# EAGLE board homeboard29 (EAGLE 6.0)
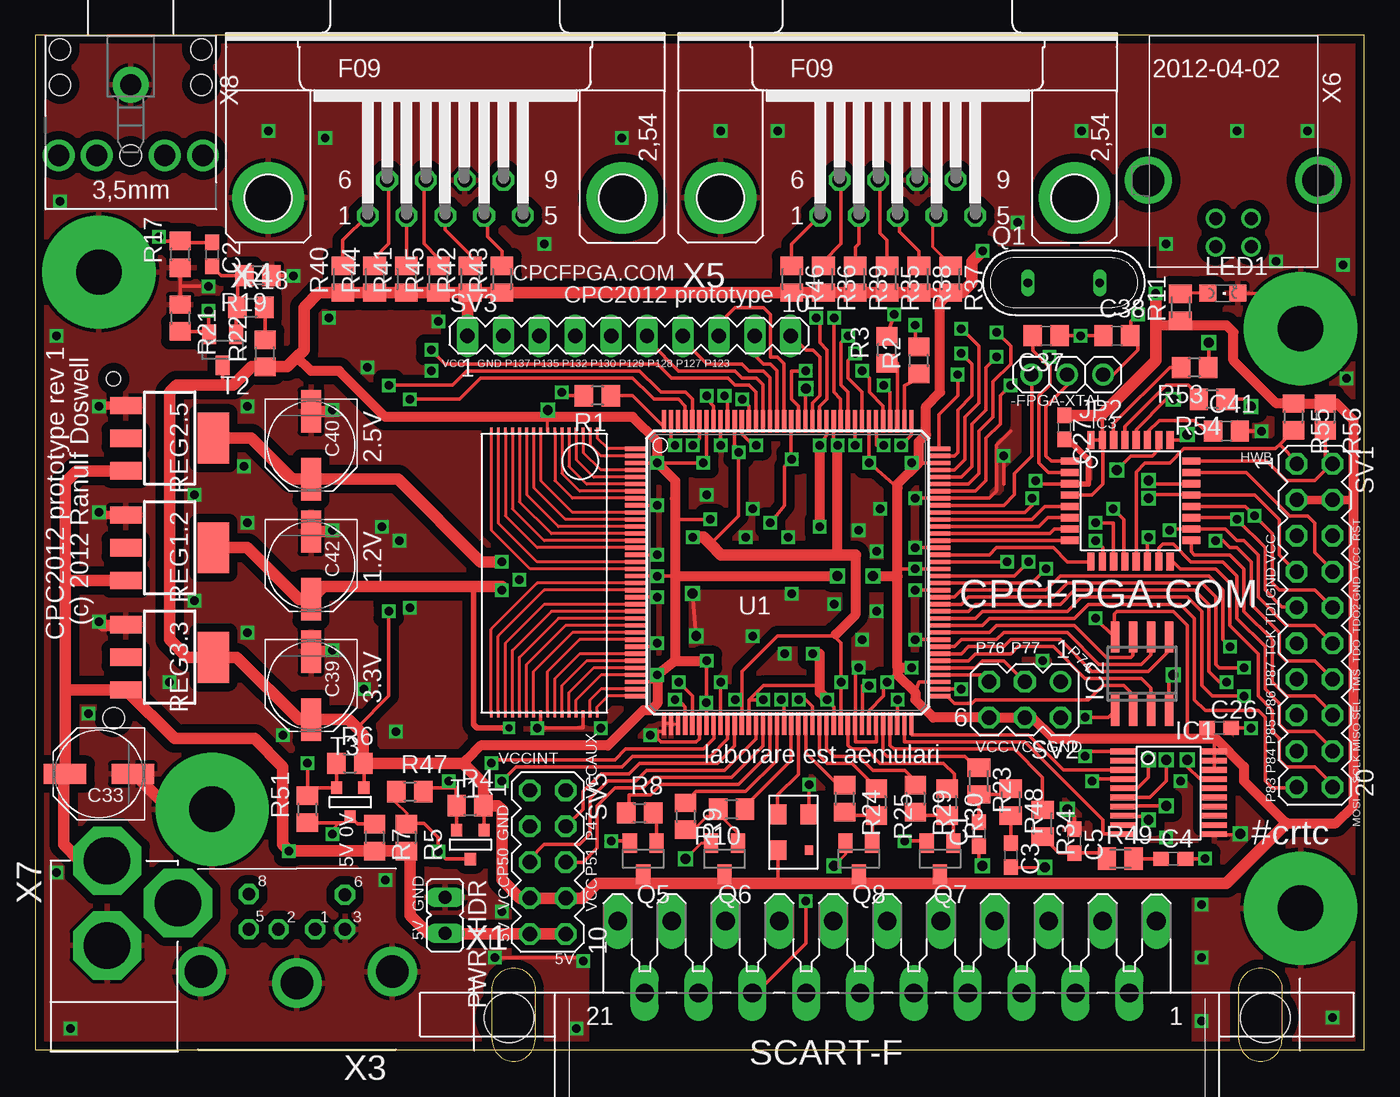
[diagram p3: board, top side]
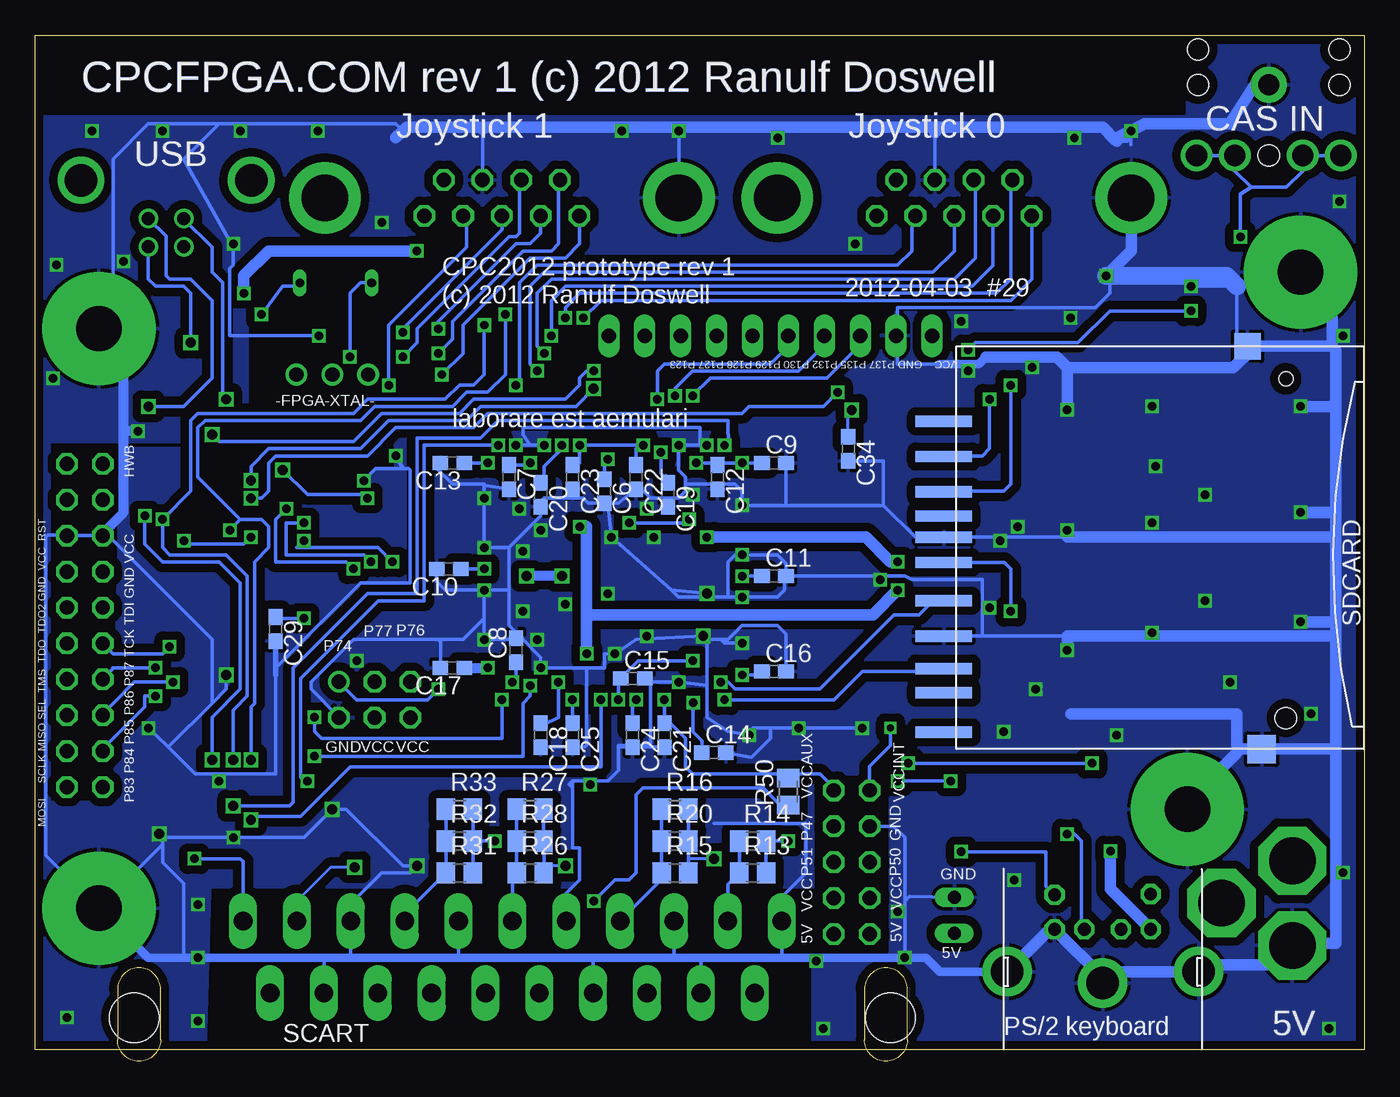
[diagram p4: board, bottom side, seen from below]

Size 94 x 72.58 mm. Coordinates in mm from the lower left corner, seen from the top.
Outline: 0,0.83 94,0.83 94,72.58 0,72.58 0,0.83
Copper layers (1*16): Top 0.0356mm / dielectric 1.5011mm / Bottom 0.0356mm
Design rules: minimum track width 7mil, minimum drill 15mil, track to track 7mil, track to pad 7mil, pad to pad 7mil, via to via 7mil, smd to smd 7mil, copper to edge 15mil, drill to drill 15mil, minimum pad ring 7mil, minimum via ring 7mil, stop-mask expansion 4mil, vias tented up to drill 0mil, thermal gap 10mil
Net classes: 1 power: width 0.6 mm, drill 1.1 mm, clearance 0.4 mm; 2 gnd: width 0.305 mm, drill 0.508 mm, clearance 0.152 mm

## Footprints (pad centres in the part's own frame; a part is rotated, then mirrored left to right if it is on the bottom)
C0603 = smd 1.1 x 1: 1 -0.85,0; 2 0.85,0
PANASONIC_D = smd 3 x 1.4: + 2.4,0; - -2.4,0
C0805 = smd 1.3 x 1.5: 1 -0.95,0; 2 0.95,0
VO20 = smd 0.4 x 1.8: 1 5.85,6.15; 2 5.2,6.15; 3 4.55,6.15; 4 3.9,6.15; 5 3.25,6.15; 6 2.6,6.15; 7 1.95,6.15; 8 1.3,6.15; 9 0.65,6.15; 10 0,6.15; 11 0,-0.3; 12 0.65,-0.3; 13 1.3,-0.3; 14 1.95,-0.3; 15 2.6,-0.3; 16 3.25,-0.3; 17 3.9,-0.3; 18 4.55,-0.3; 19 5.2,-0.3; 20 5.85,-0.3
SO-08 = smd 0.6 x 2.2: 1 -1.905,-2.6; 2 -0.635,-2.6; 3 0.635,-2.6; 4 1.905,-2.6; 5 1.905,2.6; 6 0.635,2.6; 7 -0.635,2.6; 8 -1.905,2.6
TQFP32-08 = smd 1.27 x 0.508: 1 -4.293,2.8; 2 -4.293,2; 3 -4.293,1.2; 4 -4.293,0.4; 5 -4.293,-0.4; 6 -4.293,-1.2; 7 -4.293,-2; 8 -4.293,-2.8; 17 4.293,-2.8; 18 4.293,-2; 19 4.293,-1.2; 20 4.293,-0.4; 21 4.293,0.4; 22 4.293,1.2; 23 4.293,2; 24 4.293,2.8 | smd 0.508 x 1.27: 9 -2.8,-4.293; 10 -2,-4.293; 11 -1.2,-4.293; 12 -0.4,-4.293; 13 0.4,-4.293; 14 1.2,-4.293; 15 2,-4.293; 16 2.8,-4.293; 25 2.8,4.293; 26 2,4.293; 27 1.2,4.293; 28 0.4,4.293; 29 -0.4,4.293; 30 -1.2,4.293; 31 -2,4.293; 32 -2.8,4.293
1X03 = drill 1.016: 1 -2.54,0; 2 0,0; 3 2.54,0
CHIPLED_0805 = smd 1.2 x 1.2: A 0,-1.05; C 0,1.05
JP1 = drill 0.914 long: 1 0,-1.27; 2 0,1.27
QS = drill 0.61 long: 1 -2.54,0; 2 2.54,0
SOT23 = smd 1 x 1.4: 1 -0.95,-1.1; 2 0.95,-1.1; 3 0,1.1
R0805 = smd 1.3 x 1.5: 1 -0.95,0; 2 0.95,0
M0805 = smd 1.3 x 1.6: 1 -0.95,0; 2 0.95,0
SOT223 = smd 1.219 x 2.235: 1 -2.311,-3.099; 2 0,-3.099; 3 2.311,-3.099 | smd 3.6 x 2.2: 4 0,3.099
MA10-2 = drill 1.016 octagon: 1 -11.43,-1.27; 2 -11.43,1.27; 3 -8.89,-1.27; 4 -8.89,1.27; 5 -6.35,-1.27; 6 -6.35,1.27; 7 -3.81,-1.27; 8 -3.81,1.27; 9 -1.27,-1.27; 10 -1.27,1.27; 11 1.27,-1.27; 12 1.27,1.27; 13 3.81,-1.27; 14 3.81,1.27; 15 6.35,-1.27; 16 6.35,1.27; 17 8.89,-1.27; 18 8.89,1.27; 19 11.43,-1.27; 20 11.43,1.27
MA03-2 = drill 1.016: 1 -2.54,-1.27 | drill 1.016 octagon: 2 -2.54,1.27; 3 0,-1.27; 4 0,1.27; 5 2.54,-1.27; 6 2.54,1.27
MA10-1 = drill 1.016 long: 1 -11.43,0; 2 -8.89,0; 3 -6.35,0; 4 -3.81,0; 5 -1.27,0; 6 1.27,0; 7 3.81,0; 8 6.35,0; 9 8.89,0; 10 11.43,0
MA05-2 = drill 1.016 octagon: 1 -5.08,-1.27; 2 -5.08,1.27; 3 -2.54,-1.27; 4 -2.54,1.27; 5 0,-1.27; 6 0,1.27; 7 2.54,-1.27; 8 2.54,1.27; 9 5.08,-1.27; 10 5.08,1.27
SOT-23 = smd 0.787 x 0.889: 1 0.025,-1.016; 2 -0.94,1.016; 3 0.991,1.016
TQ144 = smd 1.6 x 0.3: P1 -10.7,8.75; P2 -10.7,8.25; P3 -10.7,7.75; P4 -10.7,7.25; P5 -10.7,6.75; P6 -10.7,6.25; P7 -10.7,5.75; P8 -10.7,5.25; P9 -10.7,4.75; P10 -10.7,4.25; P11 -10.7,3.75; P12 -10.7,3.25; P13 -10.7,2.75; P14 -10.7,2.25; P15 -10.7,1.75; P16 -10.7,1.25; P17 -10.7,0.75; P18 -10.7,0.25; P19 -10.7,-0.25; P20 -10.7,-0.75; P21 -10.7,-1.25; P22 -10.7,-1.75; P23 -10.7,-2.25; P24 -10.7,-2.75; P25 -10.7,-3.25; P26 -10.7,-3.75; P27 -10.7,-4.25; P28 -10.7,-4.75; P29 -10.7,-5.25; P30 -10.7,-5.75; P31 -10.7,-6.25; P32 -10.7,-6.75; P33 -10.7,-7.25; P34 -10.7,-7.75; P35 -10.7,-8.25; P36 -10.7,-8.75; P73 10.7,-8.75; P74 10.7,-8.25; P75 10.7,-7.75; P76 10.7,-7.25; P77 10.7,-6.75; P78 10.7,-6.25; P79 10.7,-5.75; P80 10.7,-5.25; P81 10.7,-4.75; P82 10.7,-4.25; P83 10.7,-3.75; P84 10.7,-3.25; P85 10.7,-2.75; P86 10.7,-2.25; P87 10.7,-1.75; P88 10.7,-1.25; P89 10.7,-0.75; P90 10.7,-0.25; P91 10.7,0.25; P92 10.7,0.75; P93 10.7,1.25; P94 10.7,1.75; P95 10.7,2.25; P96 10.7,2.75; P97 10.7,3.25; P98 10.7,3.75; P99 10.7,4.25; P100 10.7,4.75; P101 10.7,5.25; P102 10.7,5.75; P103 10.7,6.25; P104 10.7,6.75; P105 10.7,7.25; P106 10.7,7.75; P107 10.7,8.25; P108 10.7,8.75 | smd 0.3 x 1.6: P37 -8.75,-10.7; P38 -8.25,-10.7; P39 -7.75,-10.7; P40 -7.25,-10.7; P41 -6.75,-10.7; P42 -6.25,-10.7; P43 -5.75,-10.7; P44 -5.25,-10.7; P45 -4.75,-10.7; P46 -4.25,-10.7; P47 -3.75,-10.7; P48 -3.25,-10.7; P49 -2.75,-10.7; P50 -2.25,-10.7; P51 -1.75,-10.7; P52 -1.25,-10.7; P53 -0.75,-10.7; P54 -0.25,-10.7; P55 0.25,-10.7; P56 0.75,-10.7; P57 1.25,-10.7; P58 1.75,-10.7; P59 2.25,-10.7; P60 2.75,-10.7; P61 3.25,-10.7; P62 3.75,-10.7; P63 4.25,-10.7; P64 4.75,-10.7; P65 5.25,-10.7; P66 5.75,-10.7; P67 6.25,-10.7; P68 6.75,-10.7; P69 7.25,-10.7; P70 7.75,-10.7; P71 8.25,-10.7; P72 8.75,-10.7; P109 8.75,10.7; P110 8.25,10.7; P111 7.75,10.7; P112 7.25,10.7; P113 6.75,10.7; P114 6.25,10.7; P115 5.75,10.7; P116 5.25,10.7; P117 4.75,10.7; P118 4.25,10.7; P119 3.75,10.7; P120 3.25,10.7; P121 2.75,10.7; P122 2.25,10.7; P123 1.75,10.7; P124 1.25,10.7; P125 0.75,10.7; P126 0.25,10.7; P127 -0.25,10.7; P128 -0.75,10.7; P129 -1.25,10.7; P130 -1.75,10.7; P131 -2.25,10.7; P132 -2.75,10.7; P133 -3.25,10.7; P134 -3.75,10.7; P135 -4.25,10.7; P136 -4.75,10.7; P137 -5.25,10.7; P138 -5.75,10.7; P139 -6.25,10.7; P140 -6.75,10.7; P141 -7.25,10.7; P142 -7.75,10.7; P143 -8.25,10.7; P144 -8.75,10.7
GNDHOLE = drill 3.2 pad 8: GND 0,0
OSC_7C = smd 0.7 x 0.6: ENA -1.27,-1.1 | smd 1.4 x 1.2: GND 1.27,-1.1; OUT 1.27,1.1; VDD -1.27,1.1
SDCARD-NOHOLE = smd 0.8 x 4 bottom: 1 7.8,0.99; 2 10.3,0.99; 3 13.5,0.99; 4 15.3,0.99; 5 18,0.99; 6 20.5,0.99; 7 22.8,0.99; 8 24.5,0.99; 9 5.3,0.99; CD 12,0.99; WP 27.3,0.99 | smd 2.032 x 2.032 bottom: MT1 28.5,-21.5 | smd 1.9 x 1.9 bottom: MT3 0,-20.5 | hole 1.5: 26.3,-23.21 | hole 1: 2.3,-23.21
TSOP32 = smd 0.5 x 0.2: P1 -9.75,3.75; P2 -9.75,3.25; P3 -9.75,2.75; P4 -9.75,2.25; P5 -9.75,1.75; P6 -9.75,1.25; P7 -9.75,0.75; P8 -9.75,0.25; P9 -9.75,-0.25; P10 -9.75,-0.75; P11 -9.75,-1.25; P12 -9.75,-1.75; P13 -9.75,-2.25; P14 -9.75,-2.75; P15 -9.75,-3.25; P16 -9.75,-3.75; P17 10.25,-3.75; P18 10.25,-3.25; P19 10.25,-2.75; P20 10.25,-2.25; P21 10.25,-1.75; P22 10.25,-1.25; P23 10.25,-0.75; P24 10.25,-0.25; P25 10.25,0.25; P26 10.25,0.75; P27 10.25,1.25; P28 10.25,1.75; P29 10.25,2.25; P30 10.25,2.75; P31 10.25,3.25; P32 10.25,3.75
SCART-CLIP = drill 1.321 long: 1 19.05,5.08; 2 17.145,0; 3 15.24,5.08; 4 13.335,0; 5 11.43,5.08; 6 9.525,0; 7 7.62,5.08; 8 5.715,0; 9 3.81,5.08; 10 1.905,0; 11 0,5.08; 12 -1.905,0; 13 -3.81,5.08; 14 -5.715,0; 15 -7.62,5.08; 16 -9.525,0; 17 -11.43,5.08; 18 -13.335,0; 19 -15.24,5.08; 20 -17.145,0; 21 -19.05,5.08 | hole 3.5: 26.75,-1.75; -26.75,-1.75
M_DIN6 = drill 0.9 pad 1.422 octagon: 1 -1.3,-3.75; 2 1.3,-3.75; 3 -3.4,-3.75; 5 3.4,-3.75; 6 -3.4,-6.2; 8 3.4,-6.25 | drill 2.3 pad 3.5: SH1 6.8,-0.75; SH2 0,0.05; SH3 -6.75,-0.75
F09HP = drill 1.016 octagon: 1 -5.486,-1.27; 2 -2.743,-1.27; 3 0,-1.27; 4 2.743,-1.27; 5 5.486,-1.27; 6 -4.115,1.27; 7 -1.372,1.27; 8 1.372,1.27; 9 4.115,1.27 | drill 3.302 pad 5.08: G1 -12.522,0; G2 12.522,0
85-32004-10X = drill 0.92 pad 1.27: 1 4.71,-1.25; 2 4.71,1.25; 3 2.71,1.25; 4 2.71,-1.25 | drill 2.3 pad 3: M1 0,6.02; M2 0,-6.02
DC-21MM = drill 3.302 pad 4.826 octagon: 1 -5.08,-3.353; 2 -0.076,-6.35; 3 -0.076,-0.356
20-0137 = drill 1.5 pad 2.54: 1 -5,0 | drill 1.5: 2 0,5.1; 3 0,2.4; 4 0,-2.4; 5 0,-5.1 | hole 1.5: -5,5; -5,-5; 0,0; -7.5,5; -7.5,-5

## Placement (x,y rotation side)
C1  [C0603]  66.75,16.08 90 top
C2  100nF  [C0603]  12.5,57.08 270 top
C3  [C0603]  69,14.58 270 top
C4  [C0603]  80.5,14.33 0 top
C5  [C0603]  73.5,15.58 270 top
C6  100nF  [C0603]  53.75,40.33 270 bottom
C7  100nF  [C0603]  60.5,41.33 270 bottom
C8  100nF  [C0603]  60,29.08 90 bottom
C9  100nF  [C0603]  41.75,42.33 0 bottom
C10  100nF  [C0603]  64.75,34.83 180 bottom
C11  100nF  [C0603]  41.75,34.33 0 bottom
C12  100nF  [C0603]  45.75,41.33 270 bottom
C13  100nF  [C0603]  64.5,42.33 180 bottom
C14  100nF  [C0603]  46,21.83 0 bottom
C15  100nF  [C0603]  51.75,27.08 0 bottom
C16  100nF  [C0603]  41.75,27.58 0 bottom
C17  100nF  [C0603]  64.5,27.83 180 bottom
C18  100nF  [C0603]  58.25,23.08 270 bottom
C19  100nF  [C0603]  49.25,40.08 270 bottom
C20  100nF  [C0603]  58.25,40.08 270 bottom
C21  100nF  [C0603]  49.5,23.08 270 bottom
C22  100nF  [C0603]  51.5,41.33 270 bottom
C23  100nF  [C0603]  56,41.33 270 bottom
C24  100nF  [C0603]  51.75,23.08 270 bottom
C25  100nF  [C0603]  56,23.08 270 bottom
C26  100nF  [C0603]  83.75,23.58 0 top
C27  100nF  [C0603]  72.8,44.84 270 top
C29  100nF  [C0603]  77,30.58 270 bottom
C33  100u  [PANASONIC_D]  4.5,20.33 180 top
C34  100nF  [C0603]  36.5,43.33 270 bottom
C37  [C0805]  71.5,51.33 180 top
C38  [C0805]  76.5,51.33 0 top
C39  100u  [PANASONIC_D]  19.5,26.58 270 top
C40  100u  [PANASONIC_D]  19.5,43.58 270 top
C41  1uF  [C0805]  84.25,44.58 0 top
C42  100u  [PANASONIC_D]  19.5,35.08 270 top
IC1  XCF02S  [VO20]  83.09,16.06 90 top
IC2  25LC080SN  [SO-08]  78.28,27.41 0 top
IC3  ATMEGA32U2-TQFP  [TQFP32-08]  77.47,39.65 0 top
JP2  [1X03]  73,48.58 180 top
LED1  [CHIPLED_0805]  84,54.33 270 top
PWR_HDR  [JP1]  29,10.33 180 top
Q1  [QS]  72.75,55.08 0 top
Q5  BC848SMD  [SOT23]  43,14.33 180 top
Q6  BC848SMD  [SOT23]  48.75,14.33 180 top
Q7  BC848SMD  [SOT23]  64,14.33 180 top
Q8  BC848SMD  [SOT23]  58.25,14.33 180 top
R1  100  [R0805]  39.76,47.07 180 top
R2  100  [R0805]  62.5,49.58 90 top
R3  100  [R0805]  60.25,50.33 90 top
R4  1000  [R0805]  30.75,18.08 0 top
R5  1000  [R0805]  26.25,15.83 270 top
R6  1000  [R0805]  22.25,21.08 0 top
R7  1000  [R0805]  24,15.83 270 top
R8  2200  [R0805]  42.75,17.58 0 top
R9  2200  [R0805]  46,17.33 270 top
R10  1000  [R0805]  49.25,17.83 180 top
R11  [M0805]  81,53.33 90 top
R13  680  [R0805]  43.25,13.33 0 bottom
R14  2200  [R0805]  43.25,15.58 0 bottom
R15  270  [R0805]  48.75,13.33 0 bottom
R16  680  [R0805]  48.75,17.83 0 bottom
R17  10000  [R0805]  10.25,57.08 90 top
R18  4700  [R0805]  15.25,53.33 0 top
R19  10000  [R0805]  15.75,55.58 180 top
R20  4700  [R0805]  48.75,15.58 0 bottom
R21  47000  [R0805]  10.25,52.58 270 top
R22  1000  [R0805]  16.25,50.08 90 top
R23  [M0805]  66.75,19.83 270 top
R24  2200  [R0805]  57.25,18.58 270 top
R25  1000  [R0805]  59.5,18.33 270 top
R26  270  [R0805]  59,13.33 0 bottom
R27  680  [R0805]  59,17.83 0 bottom
R28  4700  [R0805]  59,15.58 0 bottom
R29  2200  [R0805]  62.25,18.58 270 top
R30  1000  [R0805]  64.5,18.33 270 top
R31  270  [R0805]  64,13.33 0 bottom
R32  680  [R0805]  64,15.58 0 bottom
R33  4700  [R0805]  64,17.83 0 bottom
R34  [M0805]  71.25,16.83 270 top
R35  [M0805]  60.25,55.33 270 top
R36  [M0805]  55.75,55.33 270 top
R37  [M0805]  64.75,55.33 270 top
R38  [M0805]  62.5,55.33 270 top
R39  [M0805]  58,55.33 270 top
R40  [M0805]  21.75,55.33 90 top
R41  [M0805]  26.25,55.33 90 top
R42  [M0805]  30.75,55.33 90 top
R43  [M0805]  33,55.33 90 top
R44  [M0805]  24,55.33 90 top
R45  [M0805]  28.5,55.33 90 top
R46  [M0805]  53.5,55.33 270 top
R47  270  [R0805]  26.5,19.08 0 top
R48  [M0805]  69,18.33 270 top
R49  [M0805]  76.75,14.33 0 top
R50  2k2  [M0805]  40.75,19.08 90 bottom
R51  270  [R0805]  19.25,17.83 90 top
R53  22  [R0805]  82,49.08 180 top
R54  22  [R0805]  83.25,46.83 180 top
R55  4700  [R0805]  89,45.58 270 top
R56  4700  [R0805]  91.25,45.58 270 top
REG1.2  1.2V  [SOT223]  9.5,36.33 270 top
REG2.5  2.5V  [SOT223]  9.5,44.08 270 top
REG3.3  3.3V  [SOT223]  9.5,28.58 270 top
SV1  [MA10-2]  90.5,30.83 270 top
SV2  [MA03-2]  70,25.58 180 top
SV3  [MA10-1]  42,51.33 0 top
SV5  [MA05-2]  36.25,14.08 270 top
T1  BSS138  [SOT-23]  30.75,15.33 0 top
T2  BC848  [SOT23]  13.25,50.33 180 top
T3  BSS138  [SOT-23]  22.25,18.33 0 top
U1  XC3S400TQ144  [TQ144]  53.22,34.58 0 top
U$1  GNDHOLE  [GNDHOLE]  12.5,17.83 0 top
U$2  TXO_7C  [OSC_7C]  53.62,16.2 90 top
U$3  SDMMCNOHOLE  [SDCARD-NOHOLE]  28.75,50.58 270 top
U$6  AS6C4008  [TSOP32]  36,34.83 270 top
U$7  GNDHOLE  [GNDHOLE]  4.5,55.83 0 top
U$8  GNDHOLE  [GNDHOLE]  89.5,51.83 0 top
U$9  GNDHOLE  [GNDHOLE]  89.5,10.83 0 top
X1  SCART-CLIP  [SCART-CLIP]  60.25,4.83 0 top
X3  [M_DIN6]  18.5,5.58 180 top
X4  [F09HP]  29,61.08 0 top
X5  [F09HP]  61,61.08 0 top
X6  MINI-USB_4P-85-32004-10X  [85-32004-10X]  84.75,62.33 270 top
X7  DC21MMX  [DC-21MM]  5,7.83 180 top
X8  STEREOJACK  [20-0137]  6.75,64.08 270 top

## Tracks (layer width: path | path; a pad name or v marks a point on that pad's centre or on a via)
AT_CLKO  (via drill 0.7)
  Top 0.254: v78.75,41.08 79,40.83 81.74,40.83 IC3.22 | U1.P124 54.47,47.55 v54.5,47.58
  Bottom 0.254: v78.75,41.08 78.75,42.08 77.5,43.33 71,43.33 69,45.33 63.5,45.33 62.5,46.33 55.75,46.33 v54.5,47.58
AT_RESET
  Top 0.254: IC3.24 87.13,42.45 88.5,41.08 90.5,41.08 91.75,42.33 | 91.75,42.33 91.75,42.28 SV1.2 | R56.2 91.25,42.83 91.75,42.33
B0
  Top 0.254: U1.P63 57.47,22.36 57.75,22.08 58.75,22.08 59.75,21.08 64.25,21.08 65,20.33 65,19.53 R30.1
B1
  Top 0.254: U1.P60 55.97,22.11 56.5,21.58 58.25,21.58 59.25,20.58 61.5,20.58 62.25,19.83 R29.1
CASIN  (via drill 0.6)
  Top 0.254: R21.2 12.1,51.63 T2.2 12.3,51.63 12.5,51.83 12.25,51.83 v12.25,53.08 | U1.P131 50.97,47.36 50.5,47.83 49.5,47.83 49,48.33 45,48.33 44,49.33 29,49.33 v28,50.33
  Bottom 0.254: v12.25,53.08 18,53.08 20.25,50.83 27.5,50.83 v28,50.33
CLK16
  Top 0.254: U1.P56 53.97,20.3 52.5,18.83 52.5,17.5 U$2.OUT
CLK_5V  (via drill 0.6)
  Top 0.2: 26.3,16.83 26.3,17.53 25.5,18.33 25.5,19.03 R47.1
  Top 0.254: T1.1 29.02,14.31 v28.5,14.83 28.5,15.83 27.5,16.83 26.3,16.83 R5.1
  Bottom 0.254: v28.5,14.83 22.5,14.83 22.5,12.38 X3.6
CSYNC
  Top 0.254: U1.P52 51.97,21.8 49.75,19.58 44.25,19.58 43.5,18.83 42,18.83 42,17.78 R8.1
DATA_5V  (via drill 0.6)
  Top 0.2: v21,16.08 21,16.38 21.5,16.88
  Top 0.254: R7.1 22.81,16.78 T3.1 21.84,16.88 21.5,16.88 R51.1
  Bottom 0.254: v21,16.08 20.5,16.08 20,15.58 20,9.53 X3.1
EMER_BOOT
  Top 0.254: SV1.1 89.23,42.4 88.05,43.58 88.05,43.68 | 88.05,43.68 R55.2 | IC3.13 77.87,41.7 78.5,42.33 80.25,42.33 81.25,43.33 87.7,43.33 88.05,43.68
EXP_A
  Top 0.254: U1.P47 49.47,22.3 48.25,21.08 42.75,21.08 42,20.33 40,20.33 38.75,19.08 38.75,17.83 37.52,16.6 SV5.4
EXP_B
  Top 0.254: U1.P50 50.97,22.8 48.75,20.58 43.25,20.58 42.5,19.83 40.5,19.83 39.25,18.58 39.25,16.08 38.5,15.33 36,15.33 34.98,14.31 SV5.5
EXP_C
  Top 0.254: U1.P51 51.47,22.3 49.25,20.08 43.75,20.08 43,19.33 41,19.33 39.75,18.08 39.75,15.08 38.75,14.08 SV5.6
EXTCLK
  Top 0.254: U1.P100 68.5,39.33 69.25,40.08 69.25,41.58 70.5,42.83 70.5,48.58 JP2.3
FL_DI
  Top 0.254: U1.P79 65.5,28.83 66,29.33 68.5,29.33 69,29.83 72.5,29.83 74.75,27.58 78.75,27.58 80.19,29.01 IC2.5
FL_DO
  Top 0.254: IC2.2 77.64,25.93 77,26.58 75.5,26.58 74.5,25.58 66.5,25.58 66.25,25.33 65,25.33 64.5,25.83 U1.P73
FL_HOLD
  Top 0.254: U1.P82 67.5,30.33 68,30.83 73.5,30.83 75.75,28.58 77.5,28.58 77.64,28.72 IC2.7
FL_SCLK
  Top 0.254: U1.P80 65,29.33 65.5,29.83 68,29.83 68.5,30.33 73,30.33 75.25,28.08 78.25,28.08 78.92,28.74 IC2.6
FL_SEL  (via drill 0.6)
  Top 0.254: v74.25,24.33 75.89,24.33 IC2.1 | v61,25.58 61,23.91 U1.P70
  Bottom 0.254: v74.25,24.33 74.25,23.33 73.75,22.83 61,22.83 v61,25.58
FL_WP
  Top 0.254: U1.P78 66,28.33 66.5,28.83 69,28.83 69.5,29.33 72,29.33 74.25,27.08 78.25,27.08 78.92,26.41 IC2.3
FPGA_AUDIO_LEFT
  Top 0.254: U1.P68 59.97,21.86 60.25,21.58 65.75,21.58 66.55,20.78 R23.1
FPGA_AUDIO_RIGHT
  Top 0.254: U1.P69 60.47,22.36 60.75,22.08 69.25,22.08 71.25,20.08 R34.1
G0
  Top 0.254: U1.P59 55.47,21.61 56,21.08 57.75,21.08 59,19.83 R25.1
G1
  Top 0.254: U1.P57 54.5,23.85 54.5,21.83 56.75,19.58 R24.1
GND  (via drill 0.6, 0.7)
  Top 0.2: U1.P37 U1.P38 U1.P39 | IC1.11 85.24,16.06 v85.25,16.08 | LED1.C 87,54.33 U$8.GND
  Top 0.254: U1.P9 v44,39.33 | U1.P22 v44,32.83 | U1.P16 v44,35.83 | U1.P81 v62.25,29.83 | U1.P88 v62.25,33.33 | U1.P94 v62.25,36.33 | U1.P117 57.97,43.86 v58,43.58 | v60,43.58 59.5,43.58 59.5,45.33 59.47,45.3 U1.P114 | U$6.P30 38.75,23.58 35.75,23.58 | U$6.P24 35.75,23.58 | 35.75,23.58 v35.5,23.58 | 44,23.33 v43.5,23.08 | U1.P29 43.75,29.33 v44,29.58 | U1.P42 46.97,22.8 46.75,22.58 44.25,22.58 44,22.83 44,23.33 | U1.P67 59.5,23.88 59.5,22.58 58,22.58 58,23.91 | v58.25,27.83 58,27.83 58,23.91 | 58,23.91 U1.P64 | R17.1 10.25,56.08 | R21.1 10.25,54.83 | 10.25,54.83 10.25,56.08 | 10.25,56.08 10,56.33 | R19.1 v18.25,55.58 | v12.25,54.83 10.25,54.83 | v62.25,39.83 U1.P101 67.5,39.83 68,40.33 68,43.58 69,44.58 | C38.1 v73.95,51.33 C37.1 | v70.75,41.08 71,40.83 73.15,40.83 IC3.3 73.23,40.85 73.25,40.83 | U1.P37 44.47,23.86 44.5,23.83 44.5,23.33 44,23.33 | U1.P39 45.47,23.86 45.5,23.83 | 68.5,40.83 v68.5,42.83 | U1.P45 48.47,26.55 v48.5,26.83 | U1.P136 48.47,43.86 v48.5,43.58 | 7,20.33 C33.- | 46.97,45.3 U1.P139 46.97,44.05 v46.5,43.58 | U$2.GND 54.73,19.55 v54.75,19.58 | v46.75,30.08 v46.5,33.08 | C5.1 73.5,17.33 v73,17.83 | IC2.4 80.19,27.01 v80.5,27.33 | C26.2 v86,23.58 | C1.1 66.75,14.08 v67,13.83 | v86.75,44.58 85.25,44.58 | 85.25,44.58 85,44.83 | C41.2 85.25,44.58 | v32.5,7.33 38.5,7.33 v38.75,7.08
  Top 0.406: C27.2 73.09,43.99 74.5,42.58 74.5,40.83 73.25,40.83
  Top 0.6: 6,30.83 6.4,30.83 REG3.3.1
  Top 0.61: REG2.5.1 4.56,46.39 v4.5,46.33 | REG1.2.1 4.69,38.64 v4.5,38.83
  Top 0.8: C39.- 20.5,28.98 v21,29.08 | C42.- 21,37.48 v21,37.58 | C40.- 21,45.98 v21,46.08 | U$1.GND 9.5,17.83 7,20.33
  Top 0.813: 6,30.83 4.75,30.83 v4.5,31.08
  Bottom 0.2: 25.5,6.33 X3.SH3 | 22.25,9.33 X3.3 | 18.5,5.93 X3.SH2 | v85.25,16.08 85,15.83 | 85,14.08 85,14.33
  Bottom 0.254: v62.25,33.33 62.15,33.23 | 62.25,31.33 v62.25,29.83 60.1,29.83 C8.2 | 62.25,31.33 v62.25,33.33 | 47,43.58 v48.5,43.58 48.5,41.83 48,41.33 48,40.93 | 47,43.58 v46.5,43.58 | 56,39.83 55.25,39.83 54.9,39.48 C6.2 | v58,43.58 59,43.58 | 59,43.58 v60,43.58 | 34,39.33 34,42.48 C34.2 | 47,43.58 47,44.83 59.5,44.83 59.5,44.33 59,43.58 | 60.5,33.33 v62.25,33.33 | v44,32.83 45,32.83 45,35.33 44.5,35.83 v44,35.83 41.5,35.83 40.9,35.23 C11.2 32.5,34.33 32,34.08 27,34.08 27,30.08 | 60.5,36.33 v62.25,36.33 v62.25,39.83 62.25,40.83 | v35.5,23.58 42,23.58 | 42,23.58 43.25,23.58 v43.5,23.08 45,23.33 46.5,24.33 46.5,26.58 | U$3.6 27,30.08 | 27,30.08 21,30.08 | 21,37.08 U$3.3 31.75,37.08 34,39.33 | v44,29.58 45.25,29.58 45.5,29.83 | 56,19.83 56,15.08 55.5,15.08 55.5,12.83 56.5,11.83 56.44,11.77 X1.13 | v12.25,54.83 9,54.83 9,51.33 U$3.MT3 | 81,66.33 83.5,63.83 80,57.58 80,56.33 80.25,56.08 80.25,51.33 v73.95,51.33 | 81,66.33 68.5,66.33 68,65.83 | 85,15.33 85,15.83 75,15.83 v73,17.83 72,17.83 68,13.83 v67,13.83 67.5,13.33 69.5,13.33 71.68,11.15 X1.5 71.68,7.65 | 85,15.33 85,14.08 83.5,12.58 83.5,7.33 | 30,49.33 33,49.33 33,51.33 SV3.2 33,51.44 33,53.33 19,53.33 18,54.33 18,55.33 v18.25,55.58 | X5.G1 48.48,66.05 | X4.8 30.37,65.45 31,66.08 | X5.8 62.37,65.95 | 81,66.33 86,66.33 88.5,63.83 88.5,51.33 U$8.GND | 77,27.33 77,20.33 82.7,20.33 84.6,22.23 | SV2.2 72.54,24.37 74.5,26.33 74.5,26.83 71.5,29.83 65.5,29.83 | 65.5,29.83 63.75,29.83 62.25,31.33 | v70.75,41.08 69.91,41.91 68,41.91 | 68,41.91 67.59,41.91 67.5,41.83 67.5,33.83 71,33.83 77,27.83 | v68.5,42.83 68,41.91 | 52.4,22.23 C24.2 C21.2 52.65,22.23 52.75,22.33
  Bottom 0.254: 55,27.83 55,22.33 55.15,22.23 C25.2 C18.2 | 52.75,22.33 52.75,20.58 53.5,19.83 54.75,19.83 | 52.75,22.33 50.5,22.33 50.5,26.83 | C16.2 40.9,30.23 41.5,30.83 44,30.83 45,29.83 45.5,29.83 | C10.2 65.6,33.93 65,33.33 v62.25,33.33 | C17.2 65.35,29.68 65.5,29.83 | 62.25,40.83 64.5,40.83 65.6,41.93 65.6,42.23 65.5,42.33 C13.2 | C14.2 43.35,21.48 42,22.83 42,23.58 | 46.5,29.83 v46.75,30.08 51.5,29.83 v53,28.83 53.75,28.83 53.75,27.83 55,27.83 | 46.5,29.83 45.5,29.83 | C15.2 50.5,26.83 | 50.5,26.83 v48.5,26.83 46.5,26.58 | 46.5,26.58 46.5,29.83 | 41,34.33 41,33.33 41.5,32.83 48.5,32.83 49,33.33 | C9.2 40.9,39.43 41,39.33 | 41,39.33 v44,39.33 44,40.33 44.5,40.83 45.65,40.83 C12.2 46.1,40.83 47.9,40.83 48,40.93 | 34,39.33 41,39.33 | 55,27.83 v58.25,27.83 58.25,28.58 59.5,29.83 60,29.83 | C7.2 62.15,40.73 62.25,40.83 | C23.2 56,39.83 | 48,40.93 48,40.33 48.5,39.83 49.5,39.83 | 9,21.83 9,22.08 | 17.5,65.33 17.62,65.2 | SV5.3 33.29,16.62 32.5,15.83 32.5,11.33 | 32.5,11.33 v32.5,7.33 | PWR_HDR.1 32.18,11.65 32.5,11.33 | 84.6,22.23 81.5,25.33 | 81.5,25.33 80.5,26.33 v80.5,27.33 | v86,23.58 84.7,22.33 84.6,22.23 | C19.2 49.4,39.73 49.5,39.83 | v54.75,19.58 54.75,19.83 | 17.5,65.08 16.75,65.08 16.5,65.33 16.5,64.83 | 60.5,36.33 60.5,33.33 | 60.5,33.33 60.5,30.83 60,30.33 | 49.5,39.83 50.5,39.83 51.5,40.83 C22.2 52.75,39.48 C6.2 | C20.2 58.25,38.58 60.5,36.33 | 56,39.83 58,39.83 58.5,39.33 58,39.33 | 49,33.33 v53.25,37.08 53.5,39.23 C6.2 | v46.5,33.08 49,33.33 | 85,15.33 U$9.GND 93.25,14.58 93.25,37.08 93.11,37.22 91.81,37.22 SV1.6 SV1.5 | 41,7.33 41.2,7.53 X1.21 41.2,11.63 39.5,13.33 39.5,16.83 46,16.83 | X1.18 46.91,7.24 47,7.33
  Bottom 0.254: X1.17 48.82,7.51 49,7.33 | X1.14 54.53,7.29 54.5,7.33 | X1.9 64.06,7.39 64,7.33 | X1.4 73.58,7.24 73.5,7.33 | 81.5,25.33 81.5,29.83 89,37.33 | 89.25,37.33 89.25,37.08 | 54.75,19.83 56,19.83 | 56,19.83 56.25,19.58 56,19.33
  Bottom 0.406: 77,27.33 77,27.83 C29.2
  Bottom 0.6: 4.93,8.33 X7.3 | 25.5,6.33 30,6.33 31,7.33 v32.5,7.33 41,7.33 47,7.33 49,7.33 54.5,7.33 64,7.33 73.5,7.33 83.5,7.33 86,7.33 U$9.GND | 26.75,49.83 27.25,49.33 30,49.33
  Bottom 0.61: 2,36.83 2,37.08
  Bottom 0.7: 89.25,37.33 87.75,38.83 87.75,44.58 | 87.75,44.58 87.75,49.58 U$8.GND | v86.75,44.58 87.75,44.58
  Bottom 0.8: 2,30.83 2,36.83 2,38.83 | X3.SH3 22.25,9.33 | X3.3 18.5,5.93 | X3.SH2 17.7,6.33 X3.SH1 11.2,6.83 6.43,6.83 X7.3 | 30.37,65.7 30,66.08 | 30,66.08 18.5,66.08 17.62,65.2 17.5,65.08 | 2,30.08 21,30.08 v21,29.08 | 2,37.08 21,37.08 v21,37.58 | v21,46.08 21,49.08 | 7.5,22.33 7.5,22.08 9,22.08 9,24.58 20.75,24.58 | U$1.GND 12.5,18.33 9,21.83 | 2,46.33 2,50.33 2.25,50.58 | 2,46.33 2,38.83 | v4.5,46.33 2,46.33 | v4.5,38.83 2,38.83 | 2.5,31.08 2.25,31.08 2,30.83 | 2,30.83 2,30.08 | U$3.MT1 2,22.08 | 2,22.08 2,30.08 | 4.93,8.33 2,8.33 2,22.08 | U$3.MT3 2.25,50.58 | 2.25,50.58 2.25,52.58 U$7.GND | 21,49.08 9.25,49.08 8,50.33 | 26.75,49.83 21.75,49.83 21,49.08 | X4.G1 16.48,57.35 v18.25,55.58 | X8.1 7.75,69.08 9.5,66.33 15.5,66.33 17.5,65.33 | 30,66.08 31,66.08 48.5,66.08 | 48.5,66.08 62.5,66.08 | 62.5,66.08 67.75,66.08 68,65.83 68.5,65.33 | 62.37,65.95 62.5,66.08 | 48.48,66.05 48.5,66.08
  Bottom 0.813: U$3.MT1 9,22.08 | v4.5,31.08 2.5,31.08
  Bottom 1.27: v18.25,55.58 9.75,55.58 9,54.83
  other vias: 15,38.08 85,65.83 82.5,2.83 26.5,32.08 2.5,2.33 59.5,36.08 59.5,31.83 71.25,28.33 41.5,65.33 74,65.83 15,30.33 15,46.33 9.5,26.83 23.5,49.08 47.5,40.08 56.5,32.33 34.25,34.08 25.5,23.33 81,19.83 20.5,65.33 52.5,65.83 24.5,37.83 87.75,56.58 69.5,59.33 80,57.83 36,57.83 20.75,52.58 92.75,48.33 59.75,39.08 53.5,33.08 50.75,30.08 92.5,56.33 90,65.83 79.5,65.83 48.5,65.83 16.5,65.83 38.25,2.33 1.5,13.33 91.75,3.08 1.75,60.83 82.5,7.33 50.75,39.08 80,15.83 82.5,11.08 40,23.58 3.75,24.58 28,48.83 50.25,37.08 28.5,52.33 14.75,42.08 11.25,40.08 11.25,32.58 17.5,23.08 23.25,26.33 25.75,36.83 1.5,51.33 24.75,12.83 33,10.58 58.25,37.58 58.5,29.83
  pour Bottom (isolate 0.6): 0,72.83 12.5,72.83 12.5,66.83 94,66.83 94,16.33 93,16.33 93,43.83 79,43.83 79,57.33 66,57.33 66,51.33 68.5,51.33 68.5,41.83 70,41.83 71,40.83 76,40.83 76,43.33 88,43.33 88.5,12.33 56,12.33 56,19.83 54.5,19.83 54.5,26.33 53.5,26.33 53.5,19.83 51.5,19.83 51.5,12.33 39,12.33 39,20.33 0,20.33
  pour Bottom (isolate 0.6): -0.5,0.33 -0.5,23.33 33.5,23.33 33.5,7.33 39,7.33 39,0.83 82,0.83 81.5,18.33 94.5,18.33 94.5,0.83
  pour Top (isolate 0.6): 0,72.83 94.5,72.83 94.5,43.83 79.5,43.83 79.5,57.83 66.5,57.83 66.5,46.33 70,46.33 70,41.83 55.5,41.83 55.5,53.33 28.5,53.33 28.5,48.83 53.5,48.83 53.5,44.83 -0.5,44.83 -0.5,72.83
  pour Top (isolate 0.6): -0.5,1.33 -0.5,49.33 69,49.33 69,40.33 74.5,40.33 74.5,45.83 88,45.83 88,26.33 85,26.33 85,20.83 85.5,20.83 85.5,19.83 88,19.83 88,15.33 67.5,15.33 67.5,22.83 81,22.83 81,28.33 66,28.33 66,12.83 56.5,12.83 56.5,19.33 54.5,19.33 54.5,25.33 51,25.33 51,12.83 39,12.83 39,20.33 33.5,20.33 33.5,7.33 39,7.33 39,1.33
  pour Top (isolate 0.6): 94.5,0.83 94.5,17.83 82,17.83 82,0.83
HDR_MISO  (via drill 0.6)
  Top 0.254: v84.25,26.83 83.75,26.83 83,27.58 83,32.33 82,33.33 73.5,33.33 72.5,32.33 66.5,32.33 66,31.83 U1.P85
  Bottom 0.254: v84.25,26.83 87,26.83 88.5,25.33 88.97,24.83 89.23,24.57 SV1.15
HDR_MOSI
  Top 0.254: 89.07,19.4 89.25,19.58 | U1.P83 67,30.83 67.5,31.33 73.5,31.33 74.5,32.33 81,32.33 82,31.33 82,25.58 82.75,24.83 86.5,24.83 87,24.33 87,19.83 87.5,19.33 89,19.33 89.07,19.4 | SV1.19 89.07,19.4
HDR_SCLK  (via drill 0.6)
  Top 0.254: v85.5,25.83 83.25,25.83 82.5,26.58 82.5,31.83 81.5,32.83 74,32.83 73,31.83 67,31.83 66.5,31.33 U1.P84
  Bottom 0.254: v85.5,25.83 86.25,25.83 86.25,25.08 89.23,22.1 SV1.17
HDR_SEL  (via drill 0.6)
  Top 0.254: v85.5,27.83 83.75,27.83 83.5,28.08 83.5,32.83 82.5,33.83 73,33.83 72,32.83 66,32.83 65.5,32.33 U1.P86
  Bottom 0.254: v85.5,27.83 88.51,27.83 88.51,27.74 SV1.13
HDR_SPARE  (via drill 0.6)
  Top 0.254: v84.5,29.33 84,29.83 84,33.33 83,34.33 72.5,34.33 71.5,33.33 65.5,33.33 65,32.83 U1.P87
  Bottom 0.254: v84.5,29.33 85,28.83 88.5,28.83 SV1.11 89.25,29.58
JOY0_DOWN  (via drill 0.6)
  Top 0.254: U1.P118 57.47,47.36 57,47.83 57,50.83 v57.5,51.33 | R41.2 X4.2
  Bottom 0.254: v57.5,51.33 57.5,53.83 56.5,54.83 27.7,54.83 R41.2 X4.2
JOY0_FIRE1  (via drill 0.6)
  Top 0.254: U1.P116 58.47,47.36 57.5,48.33 57.5,49.58 v58,50.08 | R45.2 28.5,56.83 27.5,57.83 27.5,62.22 X4.7
  Bottom 0.254: v58,50.08 58.5,50.58 58.5,54.33 57.5,55.33 29,55.33 27.5,56.83 27.5,62.22 X4.7
JOY0_FIRE2  (via drill 0.6)
  Top 0.254: U1.P119 56.97,46.86 56.5,47.33 v56.5,52.58 | R44.2 24,56.83 25,57.83 25,62.23 X4.6
  Bottom 0.254: v56.5,52.58 56.5,53.33 55.5,54.33 26,54.33 25,55.33 25,62.23 X4.6
JOY0_LEFT  (via drill 0.6)
  Top 0.254: U1.P113 59.97,46.36 59,47.33 59,48.33 v58.5,48.83 | R42.2 30.75,57.08 29,58.83 X4.3
  Bottom 0.254: v58.5,48.83 59,49.33 59,54.83 58,55.83 30.5,55.83 29,57.33 X4.3
JOY0_RIGHT  (via drill 0.6)
  Top 0.254: U1.P112 60.47,47.36 v60,47.83 | R43.2 33,57.33 32,58.33 32,59.55 X4.4
  Bottom 0.254: v60,47.83 59.75,47.83 59.75,55.08 58.5,56.33 33,56.33 32,57.33 32,59.55 X4.4
JOY0_UP  (via drill 0.6)
  Top 0.254: U1.P122 55.47,46.3 56,46.83 56,50.33 55.5,50.83 55.5,52.33 v55.25,52.58 | R40.2 21.75,58.08 23.5,59.83 X4.1
  Bottom 0.254: v55.25,52.58 54,53.83 25,53.83 23.5,55.33 23.5,59.79 X4.1
JOY1_DOWN  (via drill 0.6)
  Top 0.254: U1.P105 65,41.83 65.75,42.58 65.75,45.58 66.75,46.58 66.75,50.58 v65.5,51.83 | R39.1 58,57.58 58.25,57.83 X5.2
  Bottom 0.254: X5.2 58.26,58.58 59.01,57.83 60,57.83 65.5,52.33 v65.5,51.83
JOY1_FIRE1  (via drill 0.6)
  Top 0.254: U1.P104 65.5,41.33 66.25,42.08 66.25,45.08 67.25,46.08 67.25,49.08 v68,49.83 | R35.1 60.25,58.08 59.75,58.58 59.75,62.22 X5.7
  Bottom 0.254: X5.7 59.75,62.22 59.75,58.58 60,58.33 60.5,58.33 67,51.83 67,50.83 v68,49.83
JOY1_FIRE2  (via drill 0.6)
  Top 0.254: R36.1 55.75,56.58 57,57.83 57,62.23 X5.6 | U1.P107 65,42.83 65.25,43.08 65.25,46.08 66.25,47.08 66.25,49.33 v65.5,50.08
  Bottom 0.254: X5.6 57,62.23 57,57.83 57.5,57.33 59.5,57.33 64.5,52.33 64.5,51.08 v65.5,50.08
JOY1_LEFT  (via drill 0.6)
  Top 0.254: U1.P103 66,40.83 66.75,41.58 66.75,44.58 67.75,45.58 67.75,48.08 69,49.33 69,50.58 v68,51.58 | R38.1 62.5,57.33 61.12,58.7 61.12,59.68 X5.3
  Bottom 0.254: 61,59.83 X5.3 61,58.83 68,51.83 v68,51.58
JOY1_RIGHT  (via drill 0.6)
  Top 0.2: R37.1 64.75,56.33 63.5,57.58 63.5,59.56 X5.4
  Top 0.254: U1.P102 66.5,40.33 67.25,41.08 67.25,44.08 68.25,45.08 68.25,47.08 v69,47.83
  Bottom 0.254: X5.4 63.5,59.56 63.5,57.58 69,52.08 v69,47.83
JOY1_UP  (via drill 0.6)
  Top 0.254: 55.5,59.83 X5.1 53.5,57.79 R46.1 | U1.P108 63.92,45.75 65.25,47.08 v65.25,48.58
  Bottom 0.254: X5.1 55.5,59.79 55.5,57.83 56.5,56.83 59,56.83 63.75,52.08 63.75,50.08 v65.25,48.58
N$1  (via drill 0.6)
  Top 0.254: U1.P135 48.97,46.86 v48.75,47.08
  Bottom 0.254: v48.75,47.08 48.75,47.58 47.5,48.83 40,48.83 38.25,50.58 38.25,51.27 SV3.4
N$2  (via drill 0.6)
  Top 0.254: U1.P132 50.47,46.36 v50,46.83
  Bottom 0.254: v50,46.83 50,48.83 49.5,49.33 42,49.33 41,50.33 41,51.08 40.75,51.33 SV3.5
N$3  (via drill 0.6)
  Top 0.254: U1.P137 47.97,46.36 47.5,46.83 v47.5,47.08
  Bottom 0.254: v47.5,47.08 46.25,48.33 38,48.33 35.5,50.83 35.5,51.18 SV3.3
N$4
  Top 0.254: U1.P130 51.47,47.86 51,48.33 50,48.33 49.5,48.83 45.5,48.83 43.5,50.83 43.5,51.1 SV3.6
N$5
  Top 0.254: U1.P129 51.97,48.36 51.5,48.83 50.5,48.83 50,49.33 47.5,49.33 46,50.83 46,51.08 45.75,51.33 SV3.7
N$6
  Top 0.254: U1.P128 52.47,48.86 52,49.33 51.5,49.33 51,49.83 51,51.33 SV3.9
N$7
  Top 0.254: U1.P127 52.97,49.36 52.5,49.83 52,49.83 52,52.83 51.5,53.33 49.5,53.33 48.5,52.33 48.5,51.48 SV3.8
N$8
  Top 0.254: 72.88,42.45 IC3.1 71.88,42.45 71.5,42.83 71.5,46.33 73,47.83 JP2.2
N$9
  Top 0.254: IC3.27 78.67,44.5 79.5,45.33 82,45.33 82.75,44.58 C41.1
N$10
  Top 0.2: LED1.A 81,54.33 R11.2
N$12  (via drill 0.6)
  Top 0.254: v71.75,49.83 71.75,49.08 | C37.2 70.55,50.28 71.75,49.08 | IC3.2 71.68,41.65 71,42.33 71,47.08 71.75,47.83 71.75,49.08
  Bottom 0.254: Q1.1 71,55.08 71.75,54.33 v71.75,49.83
N$14  (via drill 0.6)
  Top 0.254: v78,52.83 77.5,52.38 C38.2 78,51.28 78,50.33 76.25,48.58 JP2.1
  Bottom 0.254: Q1.2 75.54,54.83 76.5,54.83 v78,52.83
N$16
  Top 0.254: U1.P123 54.97,46.55 55.5,47.08 55.5,49.83 55,50.33 54.5,50.33 53.5,51.33 SV3.10
N$35
  Top 0.254: U1.P72 61.97,23.86 62,23.83 62,23.08 70.25,23.08 72.71,20.61 IC1.3
N$36  (via drill 0.7)
  Top 0.254: R53.1 83,49.13 v83,50.83
  Bottom 0.254: X6.2 86,55.33 85.5,54.83 83.5,54.83 83,54.33 v83,50.83
N$38
  Top 0.254: U1.P71 61.47,22.61 61.5,22.58 70,22.58 75.5,17.08 75.5,16.08 76.75,16.08 76.76,16.06 IC1.10
N$39
  Top 0.254: U1.P110 61.47,47.8 62.5,48.33 R2.1
N$40  (via drill 0.6, 0.7)
  Top 0.254: IC1.7 77,18.08 77,18.07 IC1.7 77.01,18.08 v80,18.08 | U1.P143 44.97,43.8 v45.25,43.58
  Bottom 0.254: v45.25,43.58 44.97,43.86 44.97,44.33 45,44.36 45,45.33 61.25,45.33 62.5,44.08 67,44.08 67,33.08 70.5,33.08 75.75,27.83 75.75,18.33 76,18.08 v80,18.08
N$42
  Top 0.254: U1.P144 44.47,44.86 42.25,47.08 40.75,47.08 40.71,47.04 | R1.1 40.71,47.04 | 40.71,47.04 40.5,46.83
N$43
  Top 0.254: U1.P111 60.97,49.41 R3.1
N$49
  Top 0.254: IC3.29 77.07,44.9 80,47.83 81.55,47.83 82.3,47.08 R54.2
N$50
  Top 0.254: REG2.5.2 6.65,44.33
N$51
  Top 0.254: C1.2 R23.2 68.6,18.88 R48.1
N$52
  Top 0.254: C3.1 R48.2
N$53
  Top 0.2: 46.3,16.38 46.55,16.38 47.5,17.33 47.8,17.33 R10.2 | 49.7,15.88 49.7,16.13 48.5,17.33 48.5,17.63
  Top 0.254: R9.2 46.3,16.38 | Q6.1 49.7,15.88 | 48.5,17.63 R10.2
N$54  (via drill 0.7)
  Top 0.2: Q6.2 47.1,15.43 v46,14.33
  Top 0.254: Q6.2 47.6,15.43
  Bottom 0.2: v46,14.33 47.8,14.33
  Bottom 0.254: R16.2 R20.2 47.8,14.33 R15.2
N$55
  Top 0.254: R24.2 57,17.38 R25.2 59.2,17.18 Q8.1
N$56  (via drill 0.7)
  Top 0.2: Q8.2 57.3,14.63 v56.5,13.83
  Top 0.254: Q8.2 57.05,14.88
  Bottom 0.2: v56.5,13.83 58,13.83
  Bottom 0.254: R27.2 R28.2 58.05,15.78 58,15.83 58,13.83 58,13.38 R26.2
N$57
  Top 0.254: Q7.1 64.95,17.08 R30.2 62.95,17.38 62.5,17.83 62.45,17.83 R29.2
N$58  (via drill 0.6)
  Top 0.254: v61.5,15.58 62.9,15.58 Q7.2
  Bottom 0.254: R31.2 R32.2 | R32.2 R33.2 | R32.2 v61.5,15.58
N$59  (via drill 0.6)
  Top 0.254: v40.75,15.58 41.65,15.58 Q5.2
  Bottom 0.254: R13.2 R14.2 v40.75,15.58
N$60
  Top 0.254: C2.2 13.15,55.58 R19.2 14.3,55.08 R18.1 14.2,53.23 T2.1
N$61  (via drill 0.6)
  Top 0.254: C2.1 9.85,57.93 R17.2 9.05,58.03 v8.75,58.33
  Bottom 0.254: 12,63.93 X8.2 X8.3 9.15,62.98 8,61.83 | X8.5 X8.4 4.35,62.98 5.5,61.83 8,61.83 | v8.75,58.33 8.75,61.33 8,61.83
N$62
  Top 0.254: R22.2 16.25,53.08 | 16.25,53.08 16.5,53.33 | R18.2 16.2,53.13 16.25,53.08
N$63
  Top 0.254: Q5.1 43.95,17.33 R8.2
N$64
  Top 0.254: C4.1 R49.2
N$65
  Top 0.254: R34.2 72.4,14.73 C5.2 75.4,14.73 R49.1
N$66  (via drill 0.7)
  Top 0.254: R54.1 85.5,46.83 v86,46.33
  Bottom 0.254: X6.3 84.75,58.37 84.75,55.58 84.5,55.33 83,55.33 81.5,53.83 81.5,48.33 83.5,46.33 v86,46.33
N$67
  Top 0.2: U$6.P1 39.75,44.08 40.5,43.33 U1.P1
N$68
  Top 0.254: IC3.30 76.27,45.1 80.25,49.08 R53.2
N$69  (via drill 0.7)
  Top 0.254: IC3.28 77.87,44.7 80,46.83 v80.5,46.83
  Bottom 0.254: v80.5,46.83 80.5,47.08 80.75,47.33 80.75,55.08 81.5,55.83 81.5,57.58 83.5,59.58 X6.4
N$71
  Top 0.2: U$6.P2 39.25,43.58 40,42.83 U1.P2
N$72
  Top 0.2: U$6.P3 38.75,43.08 40,41.83 U1.P4
N$73
  Top 0.2: U$6.P4 38.25,42.58 39.5,41.33 U1.P5
N$74
  Top 0.2: U$6.P5 37.75,42.08 39,40.83 U1.P6
N$75
  Top 0.2: U$6.P6 37.25,41.58 38.5,40.33 U1.P7
N$76
  Top 0.2: U$6.P7 36.75,41.08 38,39.83 U1.P8
N$77
  Top 0.2: U$6.P9 35.75,41.08 38,38.83 U1.P10
N$78
  Top 0.2: U$6.P10 35.25,40.58 37.5,38.33 U1.P11
N$79
  Top 0.2: U$6.P11 34.75,40.08 37,37.83 U1.P12
N$80
  Top 0.2: U$6.P12 34.25,39.58 36.5,37.33 U1.P13
N$81
  Top 0.2: U$6.P13 33.75,39.08 36,36.83 U1.P14
N$82
  Top 0.2: U$6.P14 33.25,38.58 35.5,36.33 U1.P15
N$83
  Top 0.2: U$6.P15 32.75,38.08 35.5,35.33 U1.P17
N$84
  Top 0.2: U$6.P16 32.25,37.58 35,34.83 U1.P18
N$85
  Top 0.2: U$6.P17 32.25,30.58 35.5,33.83 U1.P20
N$86
  Top 0.2: U$6.P18 32.75,30.08 36,33.33 U1.P21
N$87
  Top 0.2: U$6.P19 33.25,29.58 36,32.33 U1.P23
N$88
  Top 0.2: U$6.P20 33.75,29.08 36.5,31.83 U1.P24
N$89
  Top 0.2: U$6.P21 34.25,28.58 37,31.33 U1.P25
N$90
  Top 0.2: U$6.P22 34.75,28.08 37.5,30.83 U1.P26
N$91
  Top 0.2: U$6.P23 35.25,27.58 38,30.33 U1.P27
N$92
  Top 0.2: U$6.P25 36.25,27.58 38.5,29.83 U1.P28
N$93
  Top 0.2: U$6.P26 36.75,27.08 38.5,28.83 U1.P30
N$94
  Top 0.2: U$6.P27 37.25,26.58 39,28.33 U1.P31
N$95
  Top 0.2: U$6.P28 37.75,26.08 39.5,27.83 U1.P32
N$96
  Top 0.2: U$6.P29 38.25,25.58 40,27.33 U1.P33
N$97
  Top 0.2: U$6.P31 39.25,25.58 40,26.33 U1.P35
N$98
  Top 0.2: U$6.P32 39.75,25.08 40.5,25.83 U1.P36
PC2
  Top 0.254: U1.P98 70.5,38.33 71.42,39.25 IC3.5
PC4  (via drill 0.6, 0.7)
  Top 0.254: U1.P99 70,38.83 70.5,39.33 v70.5,39.83 | IC3.26 79.47,43.3 79,42.83 77.5,42.83 v76.5,41.83
  Bottom 0.254: v70.5,39.83 70.5,40.08 74.75,40.08 v76.5,41.83
PC5  (via drill 0.6, 0.7)
  Top 0.254: U1.P125 53.97,46.36 53.5,46.83 53.5,48.83 v54.5,48.83 | IC3.25 81.12,43.94 v81.5,44.33
  Bottom 0.254: v54.5,48.83 55,48.83 55.5,48.33 55.5,47.83 56.5,46.83 63,46.83 64,45.83 69.5,45.83 71.5,43.83 81,43.83 v81.5,44.33
PD0
  Top 0.254: U1.P97 71,37.83 71.62,38.45 IC3.6
PD1
  Top 0.254: U1.P96 71.75,37.33 72.07,37.65 IC3.7
PD2
  Top 0.254: U1.P95 73.15,36.83 IC3.8
PD3
  Top 0.254: U1.P93 67.5,35.83 68,36.33 72,36.33 73,35.33 74.64,35.33 IC3.9
PD4  (via drill 0.6)
  Top 0.254: v75,36.83 75.5,36.33 75.5,35.39 IC3.10 | U1.P92 v68.75,35.33
  Bottom 0.254: v75,36.83 75.5,36.33 69.75,36.33 v68.75,35.33
PD5  (via drill 0.6)
  Top 0.254: 76.25,35.59 IC3.11 76.25,35.34 | v75,38.08 76.25,38.08 76.25,35.34 | U1.P90 69.25,34.33 v70.25,35.33 | 76.25,35.33 76.25,35.34
  Bottom 0.254: v75,38.08 76.25,38.08 76.25,35.83 70.75,35.83 v70.25,35.33
PD6  (via drill 0.6)
  Top 0.254: v76.25,39.08 77,38.33 77,35.43 IC3.12 | U1.P89 70.5,33.83 v71.5,34.83
  Bottom 0.254: v76.25,39.08 77,38.33 77,35.33 72,35.33 v71.5,34.83
PROM_DO  (via drill 0.6)
  Top 0.254: U1.P65 58.5,23.35 58.5,26.58 v59,26.58 | IC1.1 74.59,21.91 v74.25,21.58
  Bottom 0.254: v59,26.58 59,25.83 59.5,25.33 59.5,21.58 v74.25,21.58
PROM_INITB  (via drill 0.6, 0.7)
  Top 0.254: U1.P58 54.97,25.11 54.5,25.58 v54,25.58 | v78.75,17.08 78.5,17.33 76.98,17.33 IC1.8
  Bottom 0.254: v54,25.58 54,20.83 71.75,20.83 75.25,17.33 78.5,17.33 v78.75,17.08
PS2CLK  (via drill 0.6)
  Top 0.254: U1.P46 48.97,22.8 47.75,21.58 42.25,21.58 41.5,20.83 34,20.83 v33,19.83 | v29.25,19.83 29.75,19.33 | 29.75,19.33 27.7,19.33 R47.2 | 29.75,19.33 29.75,18.13 R4.1 T1.2
  Bottom 0.254: v33,19.83 v29.25,19.83
PS2DAT  (via drill 0.6)
  Top 0.254: U1.P44 48,23.85 48,22.83 47.25,22.08 41.75,22.08 41,21.33 32.5,21.33 v32.25,21.08 | R6.1 T3.2 21.29,19.33 19.25,19.33 | R6.1 | v19.25,21.08 19.25,19.33 | 19.25,19.33 R51.2 | R6.1 20.99,21.07
  Bottom 0.254: v32.25,21.08 v19.25,21.08
R0
  Top 0.254: U1.P55 53.47,21.3 50.2,18.03 R10.1
R1
  Top 0.254: U1.P53 52.47,21.3 50.25,19.08 46.75,19.08 46,18.33 R9.1
SCART_BLANKING  (via drill 0.6)
  Top 0.254: v54.5,11.33 54.5,8.33 51.25,5.08 50.98,5.08 X1.16
  Bottom 0.254: v54.5,11.33 53,12.83 52,12.83 51.5,13.33 51.5,18.83 51,19.33 42.5,19.33 41.5,18.33 40.95,18.33 R50.1
SCART_BLUE
  Bottom 0.254: R33.1 R32.1 R31.1 67.87,10.41 X1.7
SCART_COMP
  Bottom 0.254: R14.1 R13.1 45.01,12.52 X1.19
SCART_GREEN
  Bottom 0.254: R27.1 R28.1 R26.1 60.25,13.03 X1.11
SCART_LEFT  (via drill 0.7)
  Top 0.2: C3.2 v71.4,13.73
  Bottom 0.2: v71.4,13.73 73.1,13.73 75.5,11.33
  Bottom 0.254: X1.3 75.49,11.32 75.5,11.33
SCART_RED
  Bottom 0.254: R16.1 R20.1 R15.1 50,13.03 50,12.58 52.63,9.95 X1.15
SCART_RIGHT  (via drill 0.6)
  Top 0.254: C4.2 v82.75,14.33
  Bottom 0.254: v82.75,14.33 79.5,14.33 79.3,14.13 X1.1
SD_CLK  (via drill 0.6)
  Top 0.254: U1.P41 46.5,23.88 46.5,25.83 v45.5,26.83
  Bottom 0.254: v45.5,26.83 45,26.83 44.5,26.33 38.5,26.33 33.25,31.58 31.5,31.58 30.5,32.58 U$3.5
SD_CS  (via drill 0.6)
  Top 0.254: v26.5,46.83 30,46.83 31.5,48.33 42.25,48.33 43.5,47.08 43.75,46.83 45.5,46.83 45.97,46.36 U1.P141
  Bottom 0.254: U$3.1 29.69,42.83 27,42.83 26.5,43.33 v26.5,46.83
SD_DI  (via drill 0.6)
  Top 0.254: v25,47.83 29.5,47.83 30.5,48.83 42.75,48.83 44,47.58 44.25,47.33 46,47.33 46.47,46.86 U1.P140
  Bottom 0.254: U$3.2 29.69,40.33 25.5,40.33 25,40.83 v25,47.83
SD_DO  (via drill 0.6)
  Top 0.254: U1.P40 45.97,25.05 45.75,25.33 v45.25,25.58
  Bottom 0.254: v45.25,25.58 37.5,25.58 35.5,27.58 29.94,27.58 U$3.7
SPI_MISO
  Top 0.254: IC3.17 81.76,36.06 82,35.83 84.5,35.83 85.5,34.83 85.5,31.83 87.5,29.83 87.5,26.83 88.5,25.83 90.5,25.83 91.77,24.56 SV1.16
SPI_MOSI
  Top 0.254: IC3.16 80.47,35.36 81,34.83 83.5,34.83 84.5,33.83 84.5,30.83 86.5,28.83 86.5,25.83 87.5,24.83 87.5,23.33 88,22.83 88,21.33 88.5,20.83 90.5,20.83 91.77,19.56 SV1.20
SPI_SCLK
  Top 0.254: IC3.15 79.47,36.3 79.75,36.58 80.5,36.58 81.75,35.33 84,35.33 85,34.33 85,31.33 87,29.33 87,26.33 88,25.33 88,23.83 88.5,23.33 90.5,23.33 91.77,22.06 SV1.18
SPI_SEL  (via drill 0.6)
  Top 0.254: v83.5,36.83 84,36.83 84.5,36.33 85,36.33 86,35.33 86,32.33 88,30.33 88,28.83 88.5,28.33 90.5,28.33 91.77,27.06 SV1.14 | IC3.14 78.67,37 v78.75,37.08
  Bottom 0.254: v83.5,36.83 83.5,36.58 79.25,36.58 v78.75,37.08
TCK  (via drill 0.6, 0.7)
  Top 0.254: R2.2 62.25,50.83 v62.25,52.08 | IC3.19 84.87,38.45 v85,38.33 87,36.33 87,33.33 88.19,32.14 89.19,32.14 SV1.9 | IC1.6 78.84,18.66 80,19.83 v80,21.33
  Bottom 0.254: v62.25,52.08 62.25,48.58 63,47.83 64,47.83 65,46.83 70.5,46.83 71.5,45.83 82.5,45.83 83,45.33 83,40.33 v85,38.33 85,36.33 84.5,35.83 80.5,35.83 79,34.33 79,25.83 80,24.83 v80,21.33
TDI_FPGA  (via drill 0.6, 0.7)
  Top 0.254: 39,47.08 R1.2 37.5,47.08 v37.25,47.33 | SV1.7 89.25,34.62 89.25,34.58 88,35.83 88,38.33 86.28,40.05 IC3.21 81.73,40.08 79,40.08 v78.75,39.83
  Bottom 0.254: v37.25,47.33 38.25,46.33 43.5,46.33 44,45.83 62,45.83 63,44.83 68.5,44.83 70.5,42.83 77,42.83 77.5,42.33 77.5,40.33 78,39.83 v78.75,39.83
TDO_EXP
  Top 0.254: IC3.23 85.68,41.65 88.75,38.58 90,38.58 90.5,38.08 90.5,36 91.77,34.73 SV1.8
TDO_FPGA  (via drill 0.6)
  Top 0.254: U1.P109 61.97,44.3 v61.25,43.58 | IC1.4 75.14,19.96 v74.75,19.83
  Bottom 0.254: v61.25,43.58 66.5,43.58 66.5,32.58 69.75,32.58 75.25,27.08 75.25,20.08 v74.75,19.83
TDO_PROM  (via drill 0.6, 0.7)
  Top 0.254: IC1.17 82.36,19.96 81.5,20.83 v81.5,21.33 | IC3.20 85.58,39.25 v86.25,38.58 87.5,37.33 87.5,33.83 88,33.33 90.5,33.33 91.73,32.1 SV1.10
  Bottom 0.254: v86.25,38.58 86.25,36.58 85,35.33 81,35.33 79.5,33.83 79.5,26.33 81.5,24.33 v81.5,21.33
TMS  (via drill 0.6, 0.7)
  Top 0.254: R3.2 v60.75,52.83 | v80.25,37.58 80.68,37.65 IC3.18 84.18,37.65 85,36.83 85.5,36.83 86.5,35.83 86.5,32.83 88.5,30.83 90.5,30.83 SV1.12 | v78.75,21.33 78.75,20.08 78,19.33 76.96,19.33 IC1.5
  Bottom 0.254: v60.75,52.83 60.75,48.58 62,47.33 63.5,47.33 64.5,46.33 70,46.33 71,45.33 82,45.33 82.5,44.83 82.5,41.33 79.5,38.33 | v78.75,21.33 78.75,25.08 78.5,25.33 78.5,35.33 77.5,36.33 77.5,37.83 78,38.33 79.5,38.33 | 79.5,38.33 v80.25,37.58
VCC  (via drill 0.6, 0.7)
  Top 0.2: U$6.P8 36.25,45.33 36,45.58 | v36.25,46.08 36.25,45.58 | 81,51.83 81,52.08 R11.1
  Top 0.254: T2.3 13.25,48.08 13,47.83 | T3.3 23.24,21.04 R6.2 | T1.3 31.74,18.04 R4.2 | Q5.3 43,12.58 | Q6.3 48.75,12.83 48.5,12.58 | U$2.VDD 52.52,12.6 52.5,12.58 | Q8.3 58.25,12.83 58,12.58 | Q7.3 64,12.58 | U1.P3 v44,42.33 v47.25,42.33 47.47,42.55 U1.P138 | U1.P126 53.47,42.61 v53.5,42.58 | U1.P115 58.97,42.36 v59,42.33 61,40.58 | v62,42.33 62.5,42.33 U1.P106 | U1.P91 v62.25,34.83 61,34.83 | U1.P75 62.5,26.83 62.25,26.08 | U1.P66 58.97,24.8 60,25.83 60,26.58 v60.25,26.83 60.75,27.33 61,27.33 | U1.P54 52.97,25.36 v52.75,25.58 | U1.P43 v47.47,25.36 47.47,28.3 v47.5,28.33 | U1.P34 44,26.83 | IC3.31 75.47,45.58 75.36,45.69 | IC3.4 74.72,40.05 75.5,40.83 75.5,43.91 IC3.31 | IC3.31 IC3.32 | v52,38.08 53,39.33 53,42.08 v53.5,42.58 | v47.75,38.33 45.25,38.33 45,39.83 | 53.25,42.33 v53.5,42.58 | U1.P19 v44,34.33 45.25,34.33 | v25,31.83 25,25.83 22.75,23.58 | IC2.8 76.32,30.01 | 76.32,30.01 v75,31.33 | 76.32,30.01 76.32,31.64 76.5,31.83 80.5,31.83 81.5,30.83 81.5,22.83 | IC1.18 IC1.19 IC1.20 83.39,22.72 83.5,22.83 | C26.1 82.9,22.93 83,22.83
  Top 0.6: 93.25,39.58 93.11,39.72 SV1.4 SV1.3
  Top 0.7: 45.25,34.33 45.25,38.33 45.25,41.08 v44,42.33 44,43.83 42.25,45.58 36.25,45.58 36,45.58 24.75,45.58 21.5,48.83 19.5,48.83 18.5,49.83 | 45.25,28.33 v44,27.33 44,26.83 44,25.33 43.5,24.83 43,24.83 40.5,22.33 31.5,22.33 30.5,21.33 | v62,27.83 61,27.83 | 61,27.83 61,34.33 | 61,34.33 61,34.83 61,40.58 61,40.83 62.5,42.33 62.5,43.83 63,44.33 63,46.33 64,47.33 64,53.63 R37.2 R38.2 | 61,27.83 61,27.33 62.25,26.08 62.25,25.58 63.52,24.31 SV2.6 69.98,24.31 70,24.33 | 79.25,52.08 81,52.08 84.25,52.08 84.75,51.58 84.75,49.58 87.8,46.53 R55.1 R56.1 92.05,46.53 93.25,45.33 93.25,39.58 93.25,18.08 92,16.83 88.5,16.83 85.5,19.83 85.5,20.83 83.5,22.83 83,22.83 81.5,22.83 72,22.83 70.5,24.33 70.48,24.31 SV2.4 | 45.25,28.33 v47.5,28.33 | 45.25,34.33 45.25,28.33 | 45.25,34.33 v56.75,34.33 | v59.25,34.33 61,34.33
  Top 0.813: R42.1 R45.1 R41.1 R44.1 R40.1 20.05,54.38 19,53.33 19,50.33 18.5,49.83 17.8,49.13 R22.1 15.3,49.13 14,47.83 13,47.83 10,47.83 9.5,47.33 9.5,29.83 10.75,28.58 REG3.3.4 14.25,28.58 18.65,24.18 C39.+ 22.15,24.18 22.75,23.58 23.2,23.13 R6.2 30.25,21.08 31.7,19.63 R4.2 32.75,18.08 33,17.83 33,12.83 34.29,11.54 SV5.7 SV5.8 38.71,11.54 39.75,12.58 43,12.58 48.5,12.58 52.5,12.58 58,12.58 64,12.58 84.25,12.58 88.5,16.83 | R42.1 R43.1 R46.2 R36.2 R39.2 R35.2 R38.2 | SV3.1 30.57,54.2 R42.1 | R37.2 65.55,54.38 66.25,55.08 66.25,56.58 v67,57.33 | C27.1 75.36,45.69 79.25,49.58 79.25,52.08 v79.25,54.33
  Bottom 0.2: C34.1 36.5,45.83 v36.25,46.08
  Bottom 0.25: v47.25,42.33 46.25,42.33 46,42.58
  Bottom 0.254: 42.5,42.33 C9.1 v44,42.33 45.65,42.33 C12.1 45.75,42.33 46,42.58 | v53.5,42.58 53.75,42.33 C6.1 | C7.1 59.15,42.18 v59,42.33 | v62,42.33 C13.1 | v62.25,34.83 C10.1 | C8.1 60,26.83 v60.25,26.83 | v52.75,25.58 52.75,26.68 C15.1 51.35,28.33 v47.5,28.33 | v47.47,25.36 47.47,23.3 46.85,22.68 C14.1 | v44,27.33 42.85,27.33 C16.1 | v52,38.08 48,38.08 v47.75,38.33 | C11.1 v44,34.33 | U$3.4 25.45,35.28 25,34.83 v25,31.83 | v75,31.33 77,31.33 C29.1
  Bottom 0.7: C17.1 v62,27.83 | v56.75,34.33 v59.25,34.33
  Bottom 0.813: v67,57.33 77.5,57.33 79.25,55.58 v79.25,54.33
VCC5  (via drill 0.6)
  Top 0.813: X7.2 3.15,14.18 2,15.33 2,20.23 C33.+ 2.1,26.33 | 2.1,26.33 2.1,34.33 | 2.1,34.33 2.1,40.93 2.94,41.77 REG2.5.3 | REG1.2.3 2.41,34.02 2.1,34.33 | 2.1,26.33 2.16,26.27 REG3.3.3 9.84,22.83 15.5,22.83 17.5,20.83 17.5,15.33 v17.95,14.88 R7.2 R5.2 26.5,14.63 26.5,10.33 27.77,9.06 PWR_HDR.2 29.06,9 SV5.9 SV5.10
  Bottom 0.813: v17.95,14.88 17.95,12.18 X3.5
VCCAUX  (via drill 0.6)
  Top 0.254: 50,25.58 v49.5,25.58 | U1.P62 57,23.41 v57,26.83 57,29.58 56.62,29.95 | U1.P48 50,23.41 50,25.58 | 50,25.58 50,27.58 52.5,30.08 56.5,30.08 56.62,29.95 | U1.P134 49.47,43.61 v49.75,43.08 49.75,38.58 47.75,36.58 | U1.P120 56.47,43.86 | 57,43.33 56.47,43.8 56.47,43.86 | 56.47,43.86 v56.75,43.58 | 56.5,30.33 56.62,30.2 56.62,29.95 | 56.75,36.08 57,35.83
  Top 0.7: 56.75,36.08 v56.75,43.58 | 58,35.83 58,31.58 56.62,30.2
  Top 0.813: REG2.5.4 15.25,44.08 18.15,41.18 C40.+ 25.65,41.18 31.5,35.33 v33,35.33 | v46.5,37.08 47.25,37.08 47.75,36.58 48.5,35.83 57,35.83 58,35.83
  Bottom 0.254: v49.5,25.58 C21.1 49.5,23.83 49,23.83 48,22.83 48,20.83 47.5,20.33 41,20.33 | v57,26.83 57,24.33 58,23.83 58.1,23.93 C18.1 | v56.75,43.58 56.75,43.33 58,42.08 58,41.33 58.25,41.08 C20.1 | v49.75,43.08 49.75,41.58 49.5,41.33 49.4,41.43 C19.1 | 41,20.33 40,20.33 | 40,20.33 38.5,20.33 37.5,19.33 37.52,19.31 SV5.2 | 40.3,20.28 40,20.33 | R50.2 40.75,20.58 41,20.33
  Bottom 0.813: v33,35.33 33.5,35.33 35.25,37.08 v46.5,37.08
VCCINT  (via drill 0.5, 0.6)
  Top 0.254: U1.P61 56.5,23.41 56.5,25.08 v56,25.58 | U1.P49 50.5,23.41 50.5,25.58 | 50.5,25.58 v51.5,25.58 | U1.P133 49.97,44.36 50.75,43.58 v51,43.58 | v55.5,43.58 56,44.33 56,45.33 55.97,45.3 U1.P121 | 50.5,25.58 51.5,26.58 55.5,26.58
  Top 0.406: v33.5,23.58 31.25,23.58 31,23.83 31,33.58
  Top 0.7: v56,25.58 55.5,26.08 55.5,26.58 55.5,28.83 v55,28.83 | v55.5,37.83 v55.5,43.58
  Top 0.813: REG1.2.4 15,36.33 18.65,32.68 C42.+ 20.4,33.58 31,33.58 33,33.58 v33,33.33
  Bottom 0.254: C22.1 51.5,43.33 v51,43.58 v55.5,43.58 55.5,42.33 56,41.83 C23.1 | SV5.1 34.98,20.85 33.5,22.33 v33.5,23.58 | v56,25.58 C25.1 | C24.1 51.75,25.58 v51.5,25.58
  Bottom 0.813: 55,31.58 55,37.83 v55.5,37.83 | 55,31.58 34.75,31.58 v33,33.33 | v55,28.83 55,31.58
X3
  Top 0.254: U1.P76 66.98,27.33 SV2.5
X4
  Top 0.254: U1.P77 66.5,27.83 67,28.33 68.5,28.33 70,26.83 SV2.3
X8  (via drill 0.6)
  Top 0.254: U1.P74 v65.5,26.33
  Bottom 0.254: v65.5,26.33 66.25,25.58 71.27,25.58 SV2.1

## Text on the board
Bottom: CPCFPGA.COM rev 1 (c) 2012 Ranulf Doswell
tSilk: 2012-04-02 | CPCFPGA.COM | CPC2012 prototype | CPC2012 prototype rev 1 | (c) 2012 Ranulf Doswell | VCC GND P137 P135 P132 P130 P129 P128 P127 P123 | -FPGA-XTAL- | 2.5V | HWB | 1.2V | CPCFPGA.COM | P76 | P76 | P77 | P77 | P74 | 3.3V | laborare est aemulari | VCCINT | VCC | VCC | GND | VCCAUX | P83 P84 P85 P86 P87 TCK TDI GND VCC | MOSI SCLK MISO SEL TMS TDO TDO2 GND VCC RST | GND | P47 | #crtc | VCC | P50 | P51 | GND | VCC | 5V | 5V | 5V
_tsilk: 5V 0V
_bsilk: CPCFPGA.COM rev 1 (c) 2012 Ranulf Doswell | CAS IN | Joystick 0 | Joystick 1 | USB | CPC2012 prototype rev 1 | 2012-04-03 #29 | (c) 2012 Ranulf Doswell | VCC GND P137 P135 P132 P130 P129 P128 P127 P123 | -FPGA-XTAL- | laborare est aemulari | HWB | SDCARD | P77 | P76 | P74 | VCC | VCC | GND | VCCINT | VCCAUX | P83 P84 P85 P86 P87 TCK TDI GND VCC | MOSI SCLK MISO SEL TMS TDO TDO2 GND VCC RST | GND | P47 | GND | P50 | VCC | P51 | VCC | 5V | 5V | 5V | 5V | PS/2 keyboard | SCART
